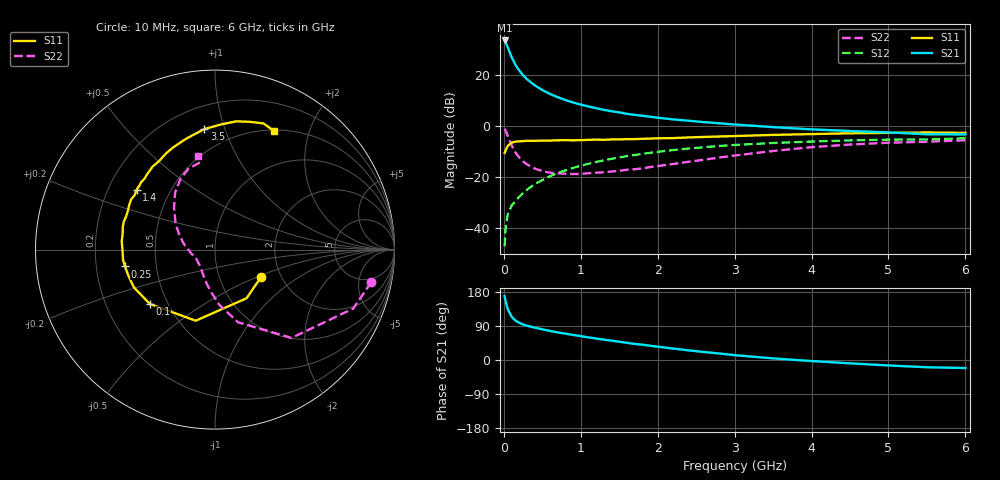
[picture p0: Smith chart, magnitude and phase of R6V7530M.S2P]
! SIEMENS Small Signal Semiconductors
! BFR193
! Si NPN RF Bipolar Junction Transistor in SOT23
! VCE = 0.75 V  IC = 30 mA
! Common Emitter S-Parameters:  May  1996
# GHz  S  MA  R  50
!  f  S11  S21  S12  S22
! GHz  MAG  ANG  MAG  ANG  MAG  ANG  MAG  ANG
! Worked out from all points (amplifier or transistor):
!   36 points, 10 MHz to 6 GHz, reference 50 ohm
!   highest |S21| = 33.5 dB at 10 MHz (marker M1)
!   |S21| within 3 dB of that: start of sweep to 54.94 MHz
!   unconditionally stable (mu >= 1): 370.5 MHz to 2.34 GHz
!   at 250 MHz: K = 0.94, MSG = 23.0 dB, |S12| = -26.2 dB
!   at 1.4 GHz: K = 1.04, MAG = 8.1 dB, |S12| = -12.8 dB
!   at 6 GHz: K = 0.99, MSG = 0.8 dB, |S12| = -4.7 dB
!   S11 on the Smith chart (normalised r, x): 10 MHz: 1.58, -0.53; 100 MHz: 0.40, -0.31; 250 MHz: 0.33, -0.08; 1.4 GHz: 0.32, +0.31; 3.5 GHz: 0.35, +0.85; 6 GHz: 0.51, +1.48
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0.01  0.299 -30.8  47.34 168.6  0.0045 80.9  0.8892 -11.8
0.02  0.3231 -57.1  45.03 158.1  0.0091 74.9  0.8374 -23.1
0.05  0.4106 -105.2  35.02 134.5  0.0187 63.7  0.651 -49.1
0.1  0.4725 -140.1  22.45 114.5  0.0276 60.4  0.4248 -72.4
0.15  0.4987 -155.1  15.9 104.2  0.0343 61.6  0.3073 -85.7
0.2  0.5043 -163.6  12.28 98.1  0.0414 64.3  0.2437 -94.1
0.25  0.5098 -169.4  9.887 93.8  0.0492 65.7  0.2048 -101.6
0.3  0.5154 -173.6  8.295 90.5  0.0569 67.5  0.1789 -107.5
0.4  0.5159 179.7  6.314 85.4  0.0731 68.7  0.149 -117.6
0.5  0.5218 174.9  5.077 81.0  0.0882 69.0  0.1315 -126.2
0.6  0.5222 170.0  4.253 76.8  0.105 68.7  0.1233 -133.0
0.7  0.5288 166.3  3.681 72.8  0.121 68.1  0.1197 -138.9
0.8  0.5316 162.8  3.232 69.5  0.1363 67.0  0.1176 -144.5
1.1  0.5393 152.3  2.423 59.7  0.1839 63.2  0.1201 -157.0
1.4  0.5494 142.7  1.954 51.1  0.23 58.7  0.1296 -167.8
1.7  0.5574 134.6  1.66 42.5  0.2726 53.9  0.1438 -178.3
2.2  0.5835 122.2  1.355 30.3  0.3404 45.5  0.1818 167.6
3  0.6396 104.2  1.077 12.8  0.429 31.8  0.266 145.8
3.5  0.6742 95.0  0.957 4.3  0.4682 23.7  0.3269 134.3
4.5  0.7243 80.6  0.803 -8.8  0.5259 9.7  0.4367 116.3
5.5  0.7531 69.0  0.693 -19.1  0.5486 -3.3  0.4957 98.8
6  0.7389 63.8  0.689 -21.2  0.5796 -7.3  0.5297 100.0
